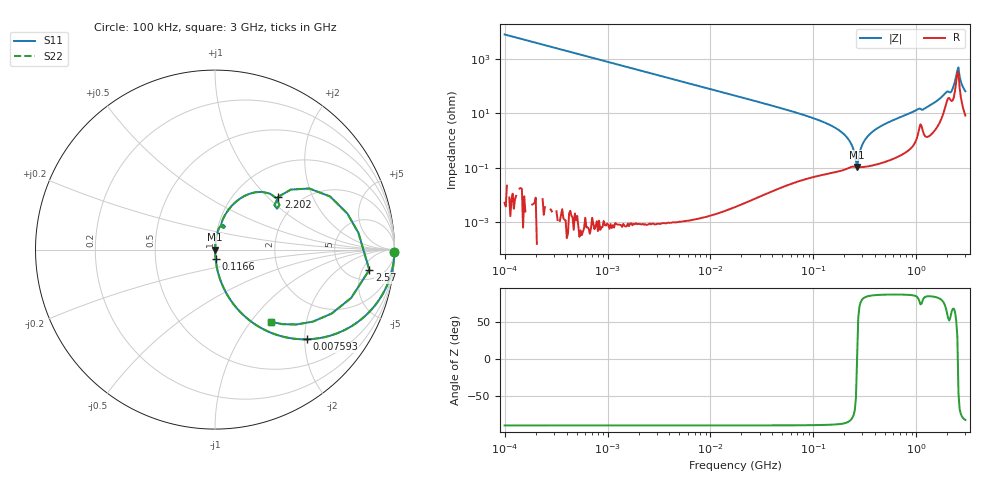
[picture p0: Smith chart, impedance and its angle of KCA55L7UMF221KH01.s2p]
!Murata Part Number: KCA55L7UMF221KH01
!These Parameters are Measured in Series Mode Connection
!Data Generated on Jan 08, 2026
!  o--ll--o
!Port1  Port2
!  o------o
!Operation Temp=25[degC], DC Bias Voltage=0[V]
!Freq. Start=100[kHz] Stop=3[GHz] 401[Steps]
# Hz S RI R 50
!Freq.(Hz) S11(Real) S11(Imag) S21(Real) S21(Imag) S12(Real) S12(Imag) S22(Real) S22(Imag)
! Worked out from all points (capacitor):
!   401 points, 100 kHz to 3 GHz, reference 50 ohm
!   read as one part in series: C = 205 pF near 105.3 kHz
!   lowest |Z| = 109 mohm at 266.1 MHz (marker M1)
!   series resonance near 265.7 MHz, so ESL is about 1.7 nH
!   S11 on the Smith chart (normalised r, x): 100 kHz: open; 7.593 MHz: 1.00, -2.04; 116.6 MHz: 1.00, -0.11; 2.202 GHz: 1.56, +1.17; 2.57 GHz: 8, -7; 3 GHz: 1.17, -1.27
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100000  0.9998 -0.0129  0.000166 0.0129  0.000166 0.0129  0.9998 -0.0129
562235  0.9948 -0.0722  0.00523 0.0722  0.00523 0.0722  0.9948 -0.0722
3161081  0.8574 -0.3497  0.1426 0.3497  0.1426 0.3497  0.8574 -0.3497
7592607  0.5099 -0.4999  0.4901 0.4999  0.4901 0.4999  0.5099 -0.4999
1.77727e7  0.1586 -0.3652  0.8414 0.3652  0.8414 0.3652  0.1586 -0.3652
9.738194e7  0.00514 -0.0683  0.9949 0.0683  0.9949 0.0683  0.00514 -0.0683
1.166348e8  0.00337 -0.0532  0.9966 0.0532  0.9966 0.0532  0.00337 -0.0532
1.630551e8  0.00156 -0.0294  0.9984 0.0294  0.9984 0.0294  0.00156 -0.0294
2.056221e8  0.00111 -0.0149  0.9989 0.0149  0.9989 0.0149  0.00111 -0.0149
2.339019e8  0.00114 -0.00731  0.9989 0.00731  0.9989 0.00731  0.00114 -0.00731
2.52704e8  0.00112 -0.0029  0.9989 0.0029  0.9989 0.0029  0.00112 -0.0029
2.660711e8  0.00108 8.62e-05  0.9989 -8.62e-05  0.9989 -8.62e-05  0.00108 8.62e-05
2.801453e8  0.00108 0.00311  0.9989 -0.00311  0.9989 -0.00311  0.00108 0.00311
3.026647e8  0.00113 0.00771  0.9989 -0.00771  0.9989 -0.00771  0.00113 0.00771
3.355313e8  0.00132 0.014  0.9987 -0.014  0.9987 -0.014  0.00132 0.014
5.475153e8  0.00421 0.0482  0.9958 -0.0482  0.9958 -0.0482  0.00421 0.0482
1.457883e9  0.0671 0.2106  0.9329 -0.2106  0.9329 -0.2106  0.0671 0.2106
2.201951e9  0.3537 0.2946  0.6463 -0.2946  0.6463 -0.2946  0.3537 0.2946
2.378954e9  0.6412 0.2961  0.3588 -0.2961  0.3588 -0.2961  0.6412 0.2961
2.570185e9  0.8597 -0.113  0.1403 0.113  0.1403 0.113  0.8597 -0.113
2.776789e9  0.5455 -0.4013  0.4545 0.4013  0.4545 0.4013  0.5455 -0.4013
3e9  0.3133 -0.4031  0.6867 0.4031  0.6867 0.4031  0.3133 -0.4031
